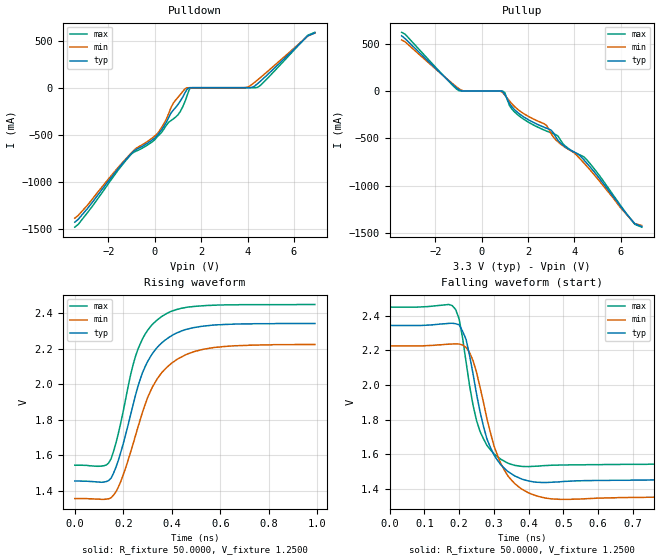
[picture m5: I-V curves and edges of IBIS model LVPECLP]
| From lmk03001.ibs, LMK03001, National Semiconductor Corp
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|   Model LVPECLP
[Model]  LVPECLP
Model_type Output
Polarity   Non-Inverting
Vmeas =  1.9400V
Rref =   50.0000
Vref =   1.2500V
C_comp   1.1000pF   1.1000pF   1.1000pF
[Temperature Range]   25.0000   85.0000   -40.0000
[Voltage Range]   3.3000V   3.1500V   3.4500V
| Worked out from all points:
|   slope of the pulldown table from 0 to 0.495 V, typ, clamps not added: 2.95 ohm
|   rising waveform, R_fixture 50.0000, V_fixture 1.2500: 20-80 % time 123ps typ, 140ps min, 104ps max; typ from 1.46 V to 2.34 V
|   falling waveform, R_fixture 50.0000, V_fixture 1.2500: 20-80 % time 61.3ps typ, 72ps min, 51.6ps max; typ from 2.34 V to 1.45 V
[Pulldown]
|Voltage   I(typ)   I(min)   I(max)
-3.45V    -1.429A    -1.387A    -1.482A
-1.1V     -722.9mA   -716.3mA   -729.3mA
100mV     -509.2mA   -491.3mA   -523.3mA
400mV     -409mA     -379.8mA   -437mA
800mV     -237.4mA   -162.8mA   -331.3mA
1V        -178mA     -102.2mA   -287.5mA
1.2V      -101.2mA   -41.1mA    -204.8mA
1.5V      -613.3uA   -58.5uA    -11.3mA
3.9V      173.5nA    754.6uA    57.2pA
4.4V      36.18mA    76.19mA    1.372mA
6.6V      551.6mA    550.5mA    558.3mA
6.9V      581.6mA    580.5mA    588.3mA
[Pullup]
|Voltage   I(typ)   I(min)   I(max)
-3.45V    581.6mA    537.7mA    618.2mA
-1V       16.83mA    27.74mA    5.801mA
900mV     -5.507mA   -15.29mA   -325.7uA
1V        -38.16mA   -43.45mA   -19.47mA
1.2V      -130.1mA   -105.9mA   -154.5mA
1.5V      -215.9mA   -182.5mA   -239.6mA
2.8V      -392.6mA   -364.2mA   -422.4mA
3.2V      -486.7mA   -515.5mA   -460.3mA
3.6V      -587.8mA   -594.2mA   -579.3mA
4.5V      -751.4mA   -783.9mA   -716.1mA
6.6V      -1.398A    -1.397A    -1.405A
6.9V      -1.428A    -1.417A    -1.435A
[Ramp]
| variable   typ   min   max
dV/dt_r  0.5335/0.1232n   0.5233/0.1420n   0.5443/0.1040n
dV/dt_f  0.5335/0.0610n   0.5220/0.0720n   0.5452/0.0514n
R_load = 50.0000
[Rising Waveform]
R_fixture= 50.0000
V_fixture= 1.2500
V_fixture_min= 1.2300
V_fixture_max= 1.2700
|time   V(typ)   V(min)   V(max)
0s        1.455V     1.356V     1.544V
140ps     1.458V     1.355V     1.557V
190ps     1.618V     1.454V     1.785V
230ps     1.827V     1.617V     2.051V
260ps     1.985V     1.756V     2.195V
300ps     2.126V     1.923V     2.302V
360ps     2.234V     2.067V     2.382V
430ps     2.293V     2.146V     2.423V
550ps     2.329V     2.201V     2.443V
990ps     2.341V     2.223V     2.448V
[Falling Waveform]
R_fixture= 50.0000
V_fixture= 1.2500
V_fixture_min= 1.2300
V_fixture_max= 1.2700
|time   V(typ)   V(min)   V(max)
0s        2.343V     2.225V     2.449V
170ps     2.355V     2.235V     2.464V
200ps     2.347V     2.236V     2.38V
220ps     2.262V     2.216V     2.131V
240ps     2.063V     2.14V      1.883V
260ps     1.847V     1.988V     1.732V
300ps     1.597V     1.65V      1.603V
340ps     1.501V     1.476V     1.549V
470ps     1.439V     1.342V     1.537V
990ps     1.454V     1.355V     1.544V
